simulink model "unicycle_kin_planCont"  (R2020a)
settings: Solver=FixedStepAuto  StartTime=0.0  StopTime=inf  FixedStep=0.01  RelTol=1e-3
model workspace (MAT data in the model file):
  SL_ROS_VariableLengthArrays_MaxSizes : object (value not decoded)
undefined symbols (not defined in the file or in its folder): Angular, cmd_vel, geometry_msgs, Linear, nav_msgs, odom, Odometry, Path, plan, Point, position_reference, Twist, X, Y
libraries: robotlib x8

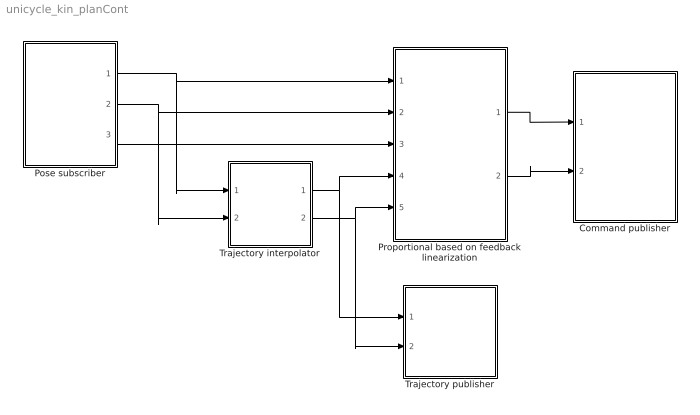
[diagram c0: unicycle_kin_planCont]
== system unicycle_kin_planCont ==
  Command publisher : Subsystem  mask{simPublishRate=50}
      mask prompts: simPublishRate "Publising rate [Hz]"
  Pose subscriber : Subsystem
  Proportional based on feedback linearization : Subsystem  mask{KP=0.5, P_dist=0.1}
      mask prompts: KP "Proportional gain"; P_dist "Point P distance"
  Trajectory interpolator : Subsystem  mask{R=0.1}
      mask prompts: R "Ball radius to switch from one point to another"
  Trajectory publisher : Subsystem  mask{simPublishRate=25}
      mask prompts: simPublishRate "Publising rate [Hz]"
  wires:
  Proportional based on feedback linearization/1(v) -> Command publisher/1(v)
  Proportional based on feedback linearization/2(w) -> Command publisher/2(w)
  Pose subscriber/1(x) -> Trajectory interpolator/1(act_x), Proportional based on feedback linearization/1(x)
  Pose subscriber/2(y) -> Trajectory interpolator/2(act_y), Proportional based on feedback linearization/2(y)
  Pose subscriber/3(theta) -> Proportional based on feedback linearization/3(theta)
  Trajectory interpolator/1(xd) -> Trajectory publisher/1(xd), Proportional based on feedback linearization/4(xd)
  Trajectory interpolator/2(yd) -> Trajectory publisher/2(yd), Proportional based on feedback linearization/5(yd)

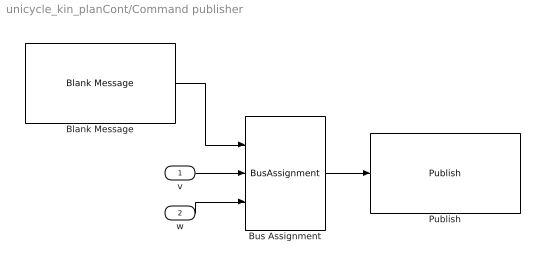
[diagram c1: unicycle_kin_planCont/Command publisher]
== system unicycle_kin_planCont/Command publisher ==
  v : Inport  SampleTime=1/simPublishRate
  w : Inport  Port=2  SampleTime=1/simPublishRate
  Blank Message : robotlib/Blank Message  messageClass=Message  entityType=geometry_msgs/Twist  messageType=geometry_msgs/Twist  SampleTime=1/simPublishRate
  Bus Assignment : BusAssignment  AssignedSignals=Linear.X,Angular.Z
  Publish : robotlib/Publish  topicSource=Specify your own  topic=/cmd_vel  messageType=geometry_msgs/Twist  messageQueueLength=1
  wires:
  Bus Assignment/1 -> Publish/1
  Blank Message/1 -> Bus Assignment/1
  v/1 -> Bus Assignment/2
  w/1 -> Bus Assignment/3

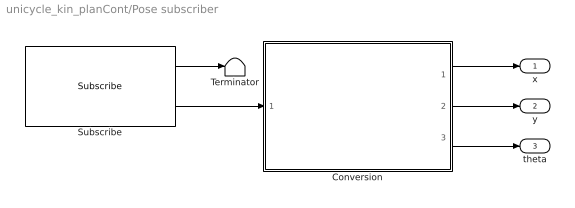
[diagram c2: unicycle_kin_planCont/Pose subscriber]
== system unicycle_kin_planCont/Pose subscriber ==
  Conversion : MATLAB Function  TreatAsAtomicUnit=on
  Subscribe : robotlib/Subscribe  topicSource=Specify your own  topic=/odom  messageType=nav_msgs/Odometry  sampleTime=-1  messageQueueLength=1
  Terminator : Terminator
  x : Outport
  y : Outport  Port=2
  theta : Outport  Port=3
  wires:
  Subscribe/1 -> Terminator/1
  Subscribe/2 -> Conversion/1(odomMsg)
  Conversion/1(x) -> x/1
  Conversion/2(y) -> y/1
  Conversion/3(theta) -> theta/1

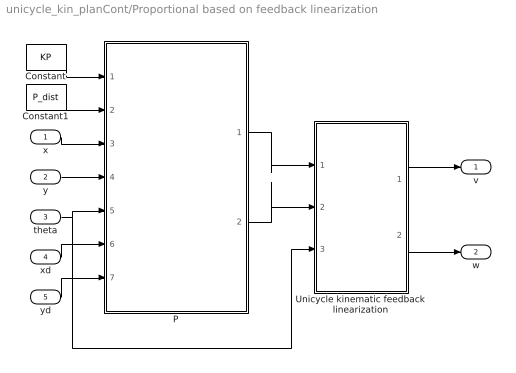
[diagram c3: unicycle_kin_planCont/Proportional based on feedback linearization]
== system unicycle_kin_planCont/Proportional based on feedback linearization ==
  x : Inport
  y : Inport  Port=2
  theta : Inport  Port=3
  xd : Inport  Port=4
  yd : Inport  Port=5
  Constant : Constant  Value=KP
  Constant1 : Constant  Value=P_dist
  P : MATLAB Function  TreatAsAtomicUnit=on
  Unicycle kinematic feedback linearization : Subsystem  mask{epsilon=0.1}
  v : Outport  VectorParamsAs1DForOutWhenUnconnected=off
  w : Outport  Port=2  VectorParamsAs1DForOutWhenUnconnected=off
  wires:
  Constant/1 -> P/1(KP)
  x/1 -> P/3(x)
  y/1 -> P/4(y)
  xd/1 -> P/6(xd)
  yd/1 -> P/7(yd)
  P/2(v_yP) -> Unicycle kinematic feedback linearization/2(v_yP)
  P/1(v_xP) -> Unicycle kinematic feedback linearization/1(v_xP)
  Unicycle kinematic feedback linearization/2(omega) -> w/1
  Unicycle kinematic feedback linearization/1(v) -> v/1
  Constant1/1 -> P/2(P_dist)
  theta/1 -> Unicycle kinematic feedback linearization/3(theta), P/5(theta)

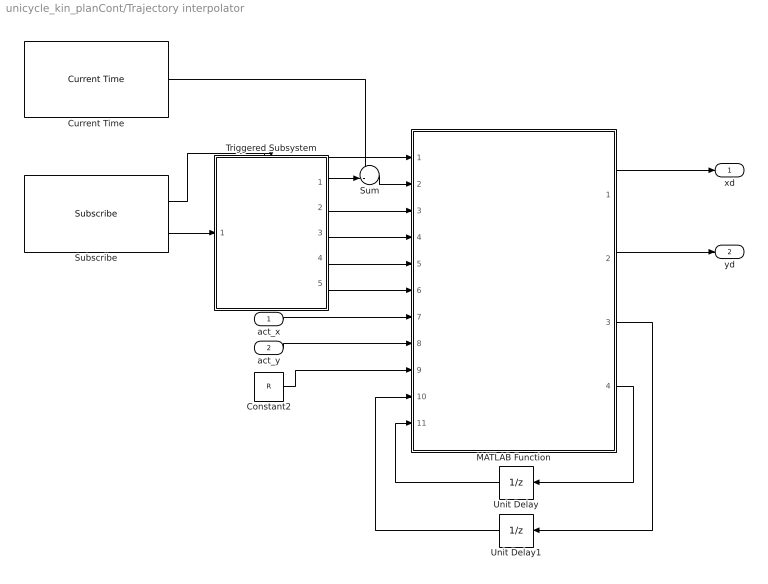
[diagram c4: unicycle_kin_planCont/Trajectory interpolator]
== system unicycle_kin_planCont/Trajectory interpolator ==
  act_x : Inport
  act_y : Inport  Port=2
  Constant2 : Constant  Value=R
  Current Time : robotlib/Current Time  OutputFormat=double  SampleTime=-1  ModelName=unicycle_kin_planCont
  MATLAB Function : MATLAB Function  TreatAsAtomicUnit=on
  Subscribe : robotlib/Subscribe  topicSource=Specify your own  topic=/plan  messageType=nav_msgs/Path  sampleTime=-1  messageQueueLength=1
  Sum : Sum  Inputs=+-|
  Triggered Subsystem : Subsystem  TreatAsAtomicUnit=on
  Unit Delay : UnitDelay  SampleTime=-1  HasFrameUpgradeWarning=on
  Unit Delay1 : UnitDelay  SampleTime=-1  HasFrameUpgradeWarning=on
  xd : Outport
  yd : Outport  Port=2
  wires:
  MATLAB Function/3(segment_idx_out) -> Unit Delay1/1
  act_x/1 -> MATLAB Function/7(act_x)
  Unit Delay1/1 -> MATLAB Function/10(segment_idx_in)
  MATLAB Function/2(plan_y) -> yd/1
  Unit Delay/1 -> MATLAB Function/11(segment_startTime_in)
  Current Time/1 -> Sum/1
  Triggered Subsystem/4(y) -> MATLAB Function/5(traj_y)
  Subscribe/2 -> Triggered Subsystem/1(path_msg)
  Triggered Subsystem/2(t) -> MATLAB Function/3(traj_t)
  Constant2/1 -> MATLAB Function/9(radius)
  MATLAB Function/4(segment_startTime_out) -> Unit Delay/1
  Triggered Subsystem/1(startTime) -> Sum/2
  act_y/1 -> MATLAB Function/8(act_y)
  MATLAB Function/1(plan_x) -> xd/1
  Triggered Subsystem/3(x) -> MATLAB Function/4(traj_x)
  Sum/1 -> MATLAB Function/2(actTime)
  Triggered Subsystem/5(numPoses) -> MATLAB Function/6(num_poses)
  Subscribe/1 -> Triggered Subsystem/Trigger, MATLAB Function/1(restart)

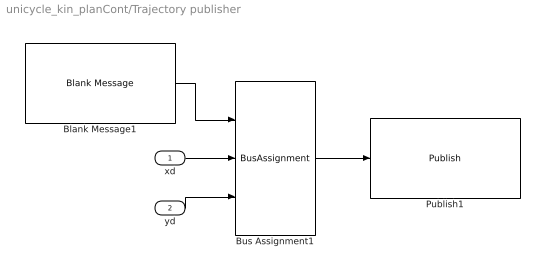
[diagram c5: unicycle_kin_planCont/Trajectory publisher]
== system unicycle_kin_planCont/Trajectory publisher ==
  xd : Inport  SampleTime=1/simPublishRate
  yd : Inport  Port=2  SampleTime=1/simPublishRate
  Blank Message1 : robotlib/Blank Message  messageClass=Message  entityType=geometry_msgs/Point  messageType=geometry_msgs/Point  SampleTime=1/simPublishRate
  Bus Assignment1 : BusAssignment  AssignedSignals=X,Y
  Publish1 : robotlib/Publish  topicSource=Specify your own  topic=/position_reference  messageType=geometry_msgs/Point  messageQueueLength=1
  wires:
  yd/1 -> Bus Assignment1/3
  xd/1 -> Bus Assignment1/2
  Blank Message1/1 -> Bus Assignment1/1
  Bus Assignment1/1 -> Publish1/1

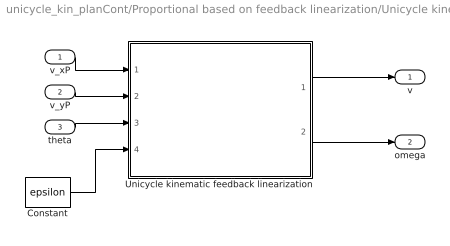
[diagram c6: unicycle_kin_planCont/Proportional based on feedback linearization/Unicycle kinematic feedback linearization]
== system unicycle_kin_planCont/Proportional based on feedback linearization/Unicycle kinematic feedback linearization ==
  v_xP : Inport
  v_yP : Inport  Port=2
  theta : Inport  Port=3
  Constant : Constant  Value=epsilon
  Unicycle kinematic feedback linearization : MATLAB Function  TreatAsAtomicUnit=on
  v : Outport  VectorParamsAs1DForOutWhenUnconnected=off
  omega : Outport  Port=2  VectorParamsAs1DForOutWhenUnconnected=off
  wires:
  Unicycle kinematic feedback linearization/2(w) -> omega/1
  v_yP/1 -> Unicycle kinematic feedback linearization/2(v_yP)
  Unicycle kinematic feedback linearization/1(v) -> v/1
  v_xP/1 -> Unicycle kinematic feedback linearization/1(v_xP)
  theta/1 -> Unicycle kinematic feedback linearization/3(theta)
  Constant/1 -> Unicycle kinematic feedback linearization/4(epsilon)

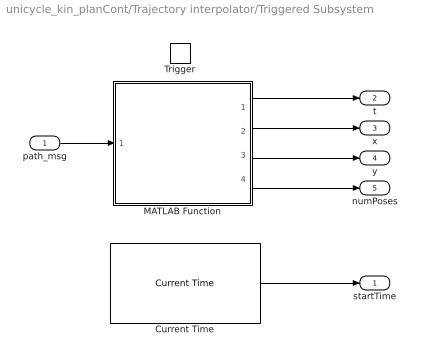
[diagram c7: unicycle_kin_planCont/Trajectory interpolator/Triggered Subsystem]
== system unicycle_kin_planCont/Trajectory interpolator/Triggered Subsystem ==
  path_msg : Inport
  Trigger : TriggerPort  VariantControl=Variant
  Current Time : robotlib/Current Time  OutputFormat=double  SampleTime=-1  ModelName=unicycle_kin_planCont
  MATLAB Function : MATLAB Function  TreatAsAtomicUnit=on
  startTime : Outport
  t : Outport  Port=2
  x : Outport  Port=3
  y : Outport  Port=4
  numPoses : Outport  Port=5
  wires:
  path_msg/1 -> MATLAB Function/1(path_msg)
  Current Time/1 -> startTime/1
  MATLAB Function/1(t) -> t/1
  MATLAB Function/3(y) -> y/1
  MATLAB Function/2(x) -> x/1
  MATLAB Function/4(num_poses) -> numPoses/1

== matlab function unicycle_kin_planCont/Proportional
based on feedback linearization/Unicycle kinematic
feedback linearization/Unicycle kinematic feedback linearization ==
function [v,w] = fblin_unicycle_kinematic(v_xP,v_yP,theta,epsilon)

v = v_xP*cos(theta)+v_yP*sin(theta);
w = (v_yP*cos(theta)-v_xP*sin(theta))/epsilon;

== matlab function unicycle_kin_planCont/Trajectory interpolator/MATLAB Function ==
function [plan_x,plan_y,segment_idx_out,segment_startTime_out] = interpolator(restart,actTime,traj_t,traj_x,traj_y,num_poses,act_x,act_y,radius,segment_idx_in,segment_startTime_in)

% Initialize input/output variables
segment_idx_out = segment_idx_in;
segment_startTime_out = segment_startTime_in;

% Start and restart logic
if (segment_idx_in==0) && (restart==0)
    plan_x = act_x;
    plan_y = act_y;
    segment_idx_out = 0;
    
    return;
end
if (restart==1)
    segment_idx_out = 1;
    segment_startTime_out = actTime;
end

% Time for trajectory interpolation
t = actTime-segment_startTime_in;

% Compute the planned point interpolating between P(idx) and P(idx+1)
if (segment_idx_out>=num_poses)
    plan_x = traj_x(num_poses);
    plan_y = traj_y(num_poses);
else
    v_x = (traj_x(segment_idx_out+1)-traj_x(segment_idx_out))/(traj_t(segment_idx_out+1)-traj_t(segment_idx_out));
    v_y = (traj_y(segment_idx_out+1)-traj_y(segment_idx_out))/(traj_t(segment_idx_out+1)-traj_t(segment_idx_out));
    
    if (v_x>=0)
        plan_x = min(traj_x(segment_idx_out)+v_x*t,traj_x(segment_idx_out+1));
    else
        plan_x = max(traj_x(segment_idx_out)+v_x*t,traj_x(segment_idx_out+1));
    end
    if (v_y>=0)
        plan_y = min(traj_y(segment_idx_out)+v_y*t,traj_y(segment_idx_out+1));
    else
        plan_y = max(traj_y(segment_idx_out)+v_y*t,traj_y(segment_idx_out+1));
    end
end

% Update the index idx
if (segment_idx_out<num_poses)
    if (sqrt((act_x-traj_x(segment_idx_out+1))^2+(act_y-traj_y(segment_idx_out+1))^2)<=radius)
        segment_idx_out = segment_idx_out+1;
        segment_startTime_out = actTime;
    end
end

== matlab function unicycle_kin_planCont/Proportional
based on feedback linearization/P ==
function [v_xP,v_yP] = P(KP,P_dist,x,y,theta,xd,yd)

% Point P transformation
xP = x+P_dist*cos(theta);
yP = y+P_dist*sin(theta);

xPd = xd+P_dist*cos(theta);
yPd = yd+P_dist*sin(theta);

% Control law
v_xP = KP*(xPd-xP);
v_yP = KP*(yPd-yP);

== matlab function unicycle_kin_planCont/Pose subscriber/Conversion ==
function [x,y,theta]  = odom_2_xytheta(odomMsg)

% Position
x = odomMsg.Pose.Pose.Position.X;
y = odomMsg.Pose.Pose.Position.Y;

% Orientation
orientation = [odomMsg.Pose.Pose.Orientation.X,odomMsg.Pose.Pose.Orientation.Y,...
    odomMsg.Pose.Pose.Orientation.Z,odomMsg.Pose.Pose.Orientation.W];

if all(orientation==zeros(1,4))
    theta = 0;
else
    eul = quat2eul(orientation,'ZYX');
    theta = eul(3);
end

== matlab function unicycle_kin_planCont/Trajectory interpolator/Triggered
Subsystem/MATLAB Function ==
function [t,x,y,num_poses]  = pathMsg2traj(path_msg)

t = zeros(1,length(path_msg.Poses));
x = zeros(1,length(path_msg.Poses));
y = zeros(1,length(path_msg.Poses));
for k=1:length(path_msg.Poses)
    t(k) = path_msg.Poses(k).Header.Stamp.Sec+path_msg.Poses(k).Header.Stamp.Nsec*1e-9;
    x(k) = path_msg.Poses(k).Pose.Position.X;
    y(k) = path_msg.Poses(k).Pose.Position.Y;
end

num_poses = path_msg.Poses_SL_Info.ReceivedLength;
